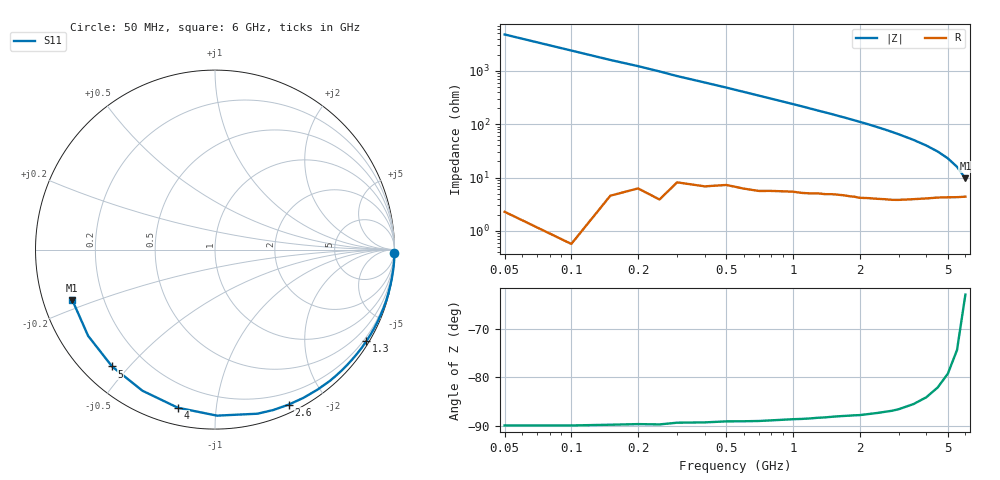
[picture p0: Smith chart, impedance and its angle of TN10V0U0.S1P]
! SIEMENS Discrete & RF Semiconductors
! BAS70-07W
! Si Schottky Diode in SOT343
! VR = 10 V
! S-Parameters:  February  1997
# GHz  S  MA  R  50
!  f  S11
! GHz  MAG  ANG
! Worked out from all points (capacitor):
!   34 points, 50 MHz to 6 GHz, reference 50 ohm
!   read as one part to ground: C = 667 fF near 50 MHz
!   lowest |Z| = 9.59 ohm at 6 GHz (marker M1)
!   S11 on the Smith chart (normalised r, x): 50 MHz: 0, -95; 1.3 GHz: 0.10, -3.58; 2.6 GHz: 0.08, -1.58; 4 GHz: 0.08, -0.79; 5 GHz: 0.09, -0.45; 6 GHz: 0.09, -0.17
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0.05  1 -1.2
0.25  0.9996 -5.9
0.3  0.9987 -7.2
0.4  0.9981 -9.5
0.6  0.9962 -14.2
0.7  0.9953 -16.6
0.8  0.9939 -19.0
0.9  0.9924 -21.4
1.1  0.9895 -26.2
1.2  0.9877 -28.7
1.3  0.9855 -31.2
1.5  0.9816 -36.0
1.6  0.9794 -38.6
1.7  0.9775 -41.0
1.8  0.9757 -43.6
1.9  0.9736 -46.1
2  0.972 -48.7
2.2  0.9669 -53.8
2.4  0.9618 -59.2
2.6  0.9562 -64.5
2.8  0.9509 -70.0
3  0.9444 -75.5
3.5  0.9252 -89.3
4  0.905 -103.2
4.5  0.8842 -117.2
5  0.8676 -131.4
5.5  0.8548 -145.8
6  0.8432 -160.5
